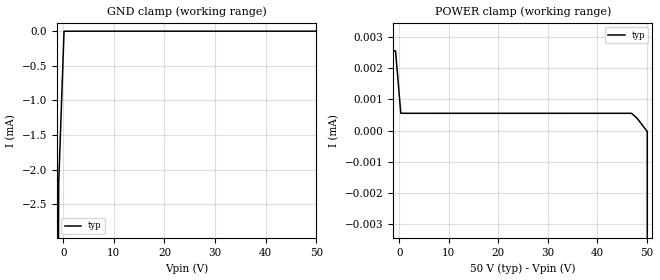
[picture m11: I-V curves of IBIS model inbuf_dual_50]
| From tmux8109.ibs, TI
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| inbuf_dual_50
[Model]   inbuf_dual_50
Model_type   Input
Vinl = 1.3
Vinh = 0.8
|   typ   min   max
C_comp   4.014581e-13   NA   NA
[Voltage Range]   50   NA   NA
[Temperature Range]   27   NA   NA
[Power Clamp Reference]   50   NA   NA
[GND Clamp Reference]   0   NA   NA
[GND Clamp]
|   Voltage   I(typ)   I(min)   I(max)
-55V      -1.557A    NA         NA
-1.97V    -30.35mA   NA         NA
-909.1mV  -2.21mA    NA         NA
151.5mV   31.08nA    NA         NA
50V       2.2uA      NA         NA
[POWER Clamp]
|   Voltage   I(typ)   I(min)   I(max)
-5V       13.2uA     NA         NA
-3.939V   2.686uA    NA         NA
-757.6mV  2.559uA    NA         NA
303mV     557.8nA    NA         NA
46.97V    554.4nA    NA         NA
48.03V    406.2nA    NA         NA
50.15V    -31.62nA   NA         NA
51.21V    -9.608mA   NA         NA
100V      -1.412A    NA         NA
